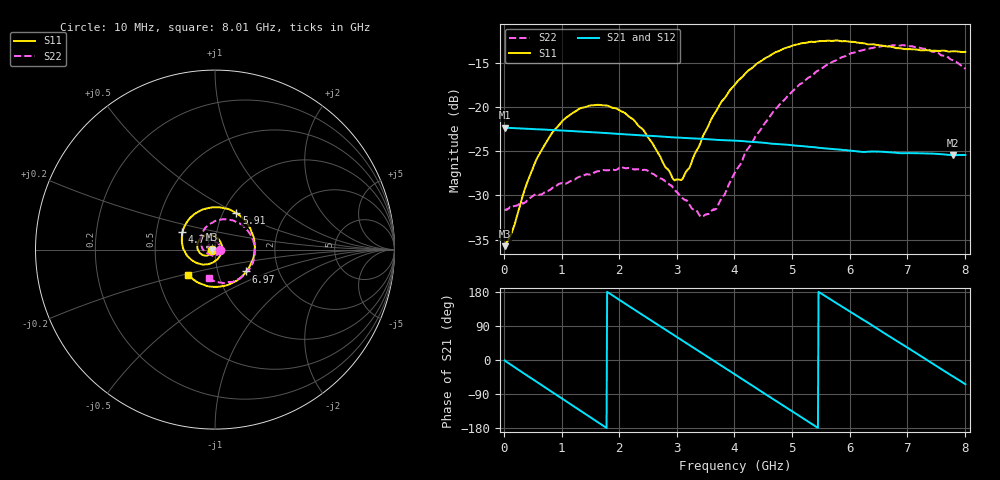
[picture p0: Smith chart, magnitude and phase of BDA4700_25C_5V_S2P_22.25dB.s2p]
!Agilent Technologies,E5071B,MY42404982,A.09.10
!Date: Mon Oct 20 13:37:35 2025
!Data & Calibration Information:
!Freq	S11:SOLT2(ON)	S21:SOLT2(ON)	S12:SOLT2(ON)	S22:SOLT2(ON)
# Hz S RI R 50
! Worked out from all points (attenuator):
!   801 points, 10 MHz to 8.01 GHz, reference 50 ohm
!   highest |S21| = -22.33 dB at 10 MHz (marker M1); lowest = -25.5 dB at 7.79 GHz (marker M2)
!   lowest |S11| = -35.8 dB at 10 MHz (marker M3), VSWR 1.03, Z = 48.4 - j0.113 ohm
!   |S11| at or under -10 dB: start of sweep to end of sweep
!   |S22| runs from -32.4 to -13.0 dB; largest |S21 - S12| = 0.00058
!   S11 on the Smith chart (normalised r, x): 10 MHz: 0.97, -0.00; 4.74 GHz: 0.68, +0.14; 5.91 GHz: 1.15, +0.50; 6.97 GHz: 1.37, -0.35; 8.01 GHz: 0.72, -0.21
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1e7  -0.0163 -0.00117  0.0765 -0.00161  0.0764 -0.00172  0.0261 -0.000828
1.4e8  -0.0175 -0.00926  0.0734 -0.0191  0.0734 -0.0192  0.0265 -0.00677
3.8e8  -0.0261 -0.0243  0.0585 -0.0473  0.0585 -0.0474  0.0213 -0.0198
6.2e8  -0.0432 -0.0335  0.0337 -0.0666  0.0337 -0.0666  0.0114 -0.0297
1.01e9  -0.0797 -0.0235  -0.0157 -0.0718  -0.0158 -0.0718  -0.0156 -0.0336
1.35e9  -0.0985 0.00928  -0.0525 -0.05  -0.0526 -0.0501  -0.0365 -0.0176
2.08e9  -0.0468 0.0806  -0.0613 0.034  -0.0614 0.034  -0.0294 0.0344
2.68e9  0.0287 0.0463  -0.00231 0.0681  -0.00235 0.0682  0.014 0.0373
2.94e9  0.0383 0.00705  0.0268 0.0617  0.0268 0.0616  0.0259 0.0233
3.09e9  0.0347 -0.0176  0.0414 0.0526  0.0412 0.0527  0.0284 0.0114
3.52e9  -0.0154 -0.0734  0.0647 0.0112  0.0648 0.0112  0.0141 -0.0202
3.7e9  -0.0514 -0.0821  0.0646 -0.00872  0.0646 -0.0089  -0.00133 -0.0271
4.01e9  -0.116 -0.067  0.0507 -0.0397  0.0507 -0.0397  -0.0333 -0.0264
4.74e9  -0.1816 0.0959  -0.0209 -0.058  -0.0207 -0.0582  -0.0805 0.0578
5.35e9  -0.061 0.2255  -0.0583 -0.0109  -0.0583 -0.0112  -0.0154 0.1497
5.91e9  0.1185 0.2037  -0.0414 0.0392  -0.0415 0.0391  0.1116 0.1577
6.27e9  0.1984 0.1133  -0.0127 0.0542  -0.0121 0.0543  0.1854 0.1009
6.68e9  0.2177 -0.0293  0.0248 0.0496  0.0249 0.0495  0.2212 -0.00179
6.97e9  0.1743 -0.1216  0.0443 0.0323  0.0444 0.032  0.207 -0.0804
7.37e9  0.058 -0.2007  0.0544 -0.00239  0.0545 -0.00247  0.1351 -0.1636
7.79e9  -0.0892 -0.1863  0.039 -0.0362  0.039 -0.0364  0.0199 -0.1829
8.01e9  -0.1488 -0.141  0.0234 -0.048  0.0235 -0.0481  -0.0331 -0.1609
